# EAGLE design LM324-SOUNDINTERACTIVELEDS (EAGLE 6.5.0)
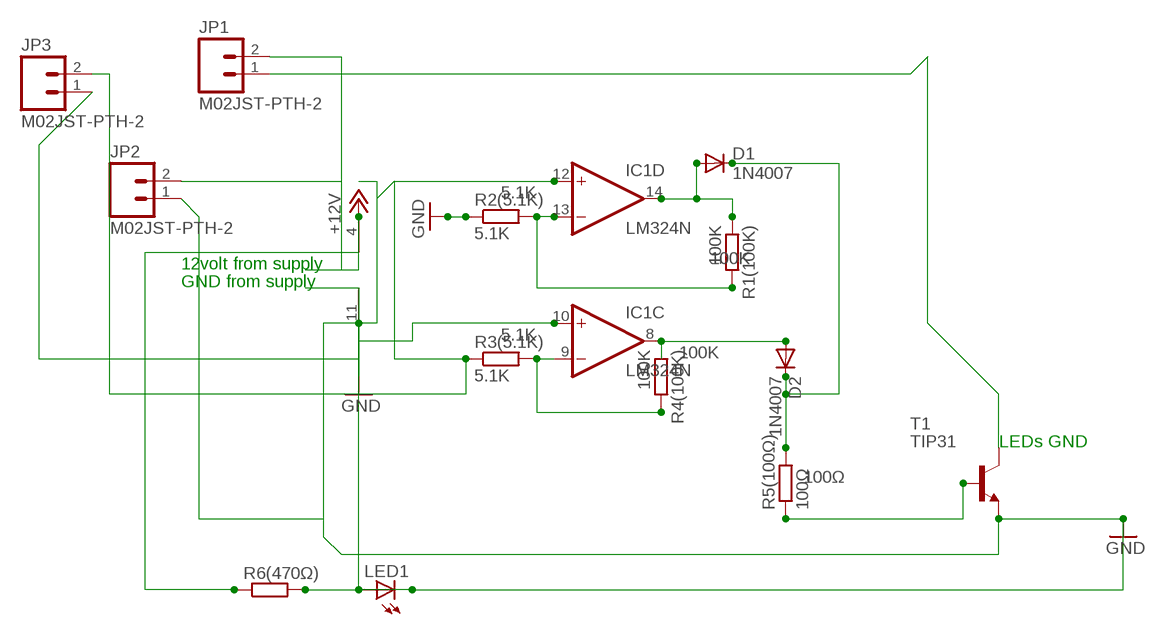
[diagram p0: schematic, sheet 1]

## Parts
D1  1N4007  1N4004  [DO41-10]
D2  1N4007  1N4004  [DO41-10]
IC1  LM324N  [DIL14]
JP1  M02JST-PTH-2  [JST-2-PTH]
JP2  M02JST-PTH-2  [JST-2-PTH]
JP3  M02JST-PTH-2  [JST-2-PTH]
LED1  LED5MM  [LED5MM]
R1(100K)  100K  R-EU_0204/7  [0204/7]
R2(5.1K)  5.1K  R-EU_0204/7  [0204/7]
R3(5.1K)  5.1K  R-EU_0204/7  [0204/7]
R4(100K)  100K  R-EU_0204/7  [0204/7]
R5(100Ω)  100Ω  R-EU_0204/7  [0204/7]
R6(470Ω)  R-EU_0204/7  [0204/7]
T1  TIP31  [TO220]

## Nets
+12V: IC1.4(P:V+) JP1.2 JP2.2 R6(470Ω).1
GND: IC1.10(C:+IN) IC1.11(P:V-) JP2.1 JP3.1 LED1.K(C) R2(5.1K).1 T1.3(E)
N$1: D1.A IC1.14(D:OUT) R1(100K).1
N$2: IC1.13(D:-IN) R1(100K).2 R2(5.1K).2
N$3: IC1.12(D:+IN) JP3.2 R3(5.1K).1
N$4: IC1.9(C:-IN) R3(5.1K).2 R4(100K).2
N$5: D2.A IC1.8(C:OUT) R4(100K).1
N$6: LED1.A R6(470Ω).2
N$7: D1.C D2.C R5(100Ω).2
N$8: JP1.1 T1.2(C)
N$11: R5(100Ω).1 T1.1(B)
Unconnected: IC1.1(A:OUT) IC1.2(A:-IN) IC1.3(A:+IN) IC1.5(B:+IN) IC1.6(B:-IN) IC1.7(B:OUT)

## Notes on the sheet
- 12volt from supply
- GND from supply
- LEDs GND

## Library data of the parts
D1 D2 = diode:1N4004: DIODE
IC1 = Unknown-5:LM324: OP AMP
JP1-JP3 = SparkFun-Connectors:M02: Standard 2-pin 0.1" header. Use with
LED1 = adafruit:LED: LED
R1(100K) = resistor:R-EU_: RESISTOR, European symbol; R1: 100K
R2(5.1K) R3(5.1K) = resistor:R-EU_: RESISTOR, European symbol; R2: 5.1K
R4(100K) = resistor:R-EU_: RESISTOR, European symbol; R4: 100K
R5(100Ω) = resistor:R-EU_: RESISTOR, European symbol; R5: 100Ω
R6(470Ω) = resistor:R-EU_: RESISTOR, European symbol
T1 = transistor:TIP31: NPN Transistor Medium Power Linear Switching Applications Source: http://onsemi.com

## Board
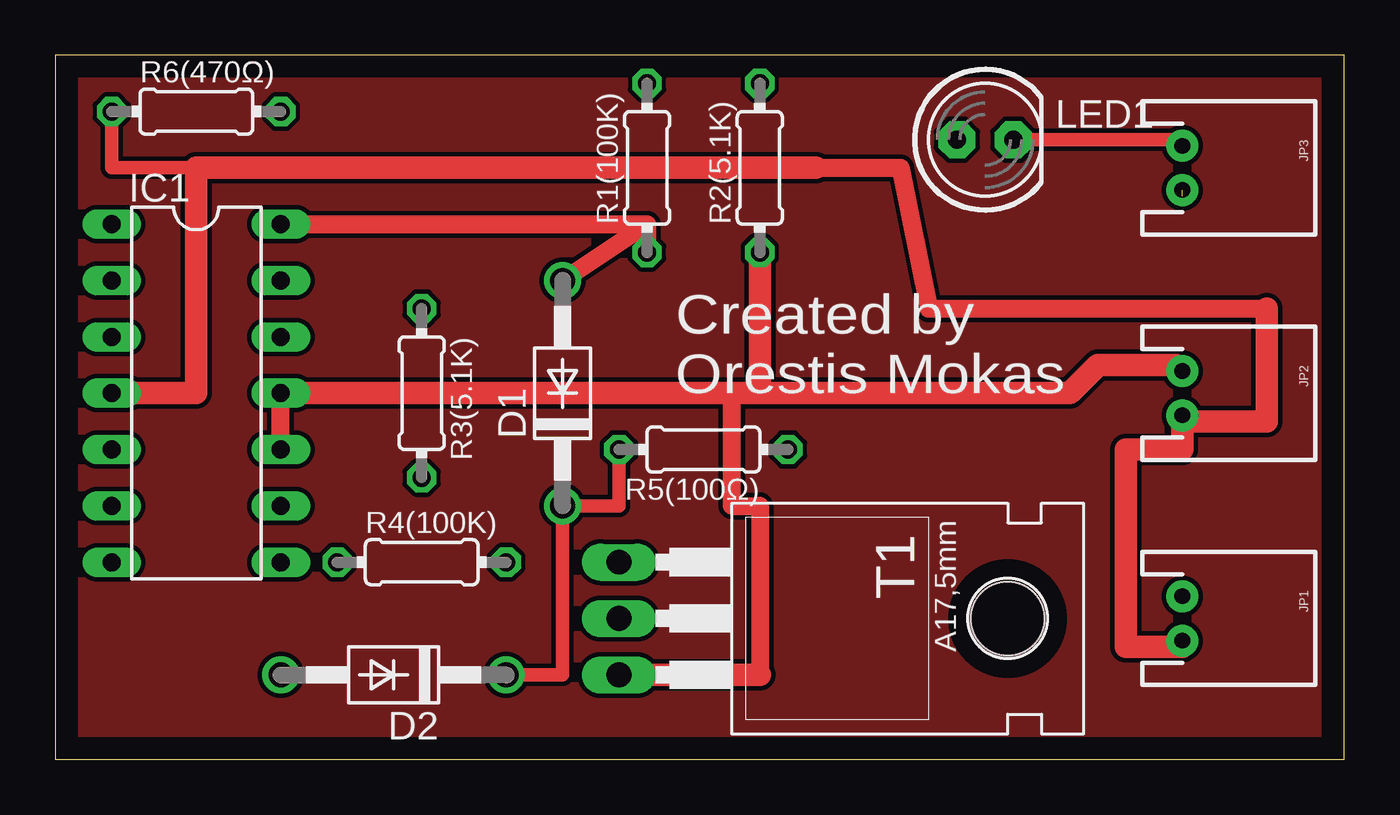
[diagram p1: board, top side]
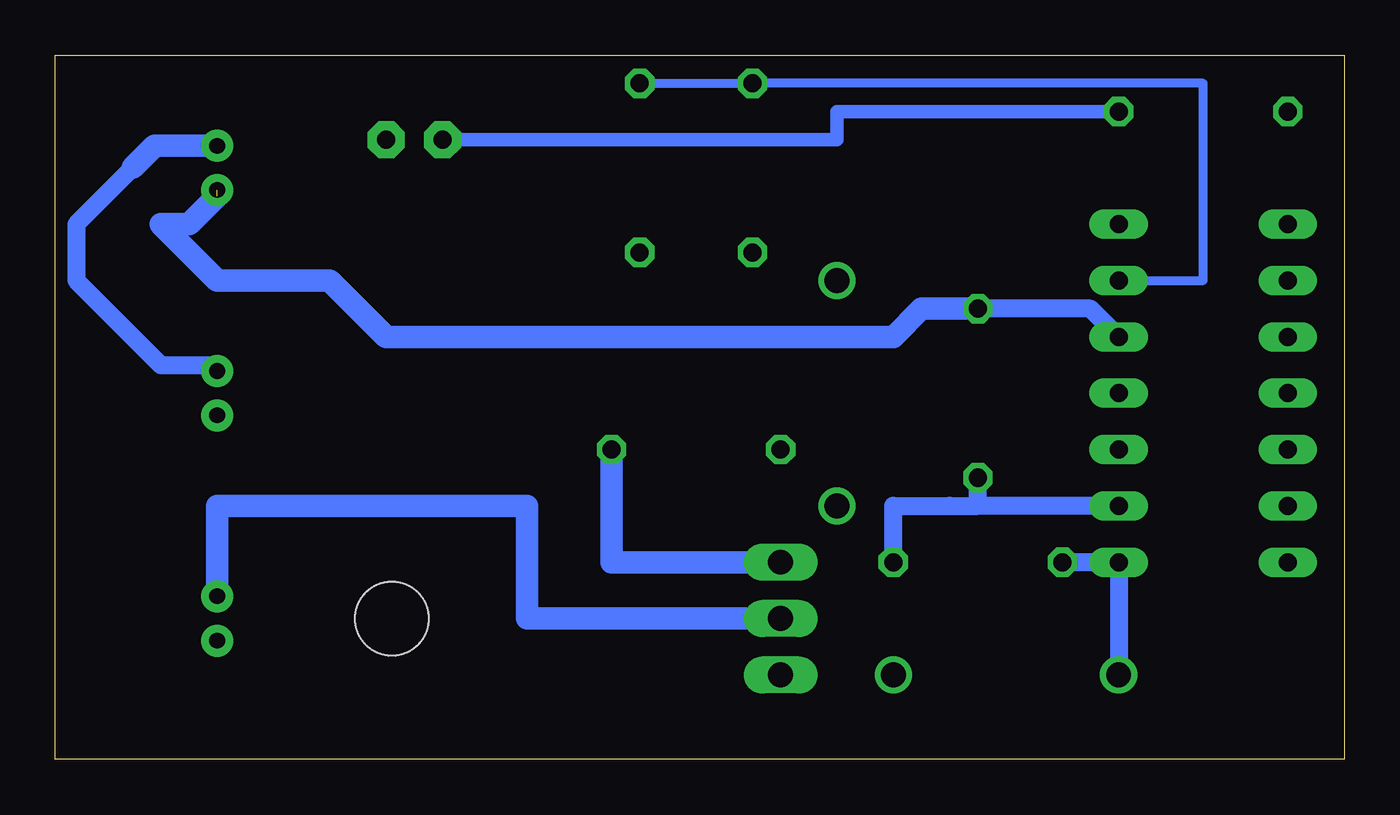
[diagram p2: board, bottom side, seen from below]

Size 58.09 x 31.74 mm. Coordinates in mm from the lower left corner, seen from the top.
Outline: 0,0 58.09,0 58.09,31.74 0,31.74 0,0
Copper layers (1*16): Top 0.035mm / dielectric 1.5mm / Bottom 0.035mm
Design rules "default": minimum track width 10mil, minimum drill 24mil, track to track 8mil, track to pad 8mil, pad to pad 8mil, via to via 8mil, smd to smd 8mil, copper to edge 40mil, drill to drill 8mil, minimum pad ring 10mil, minimum via ring 8mil, stop-mask expansion 4mil, vias tented up to drill 0mil, thermal gap 10mil

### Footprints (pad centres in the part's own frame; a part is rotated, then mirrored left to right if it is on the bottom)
DO41-10 = drill 1.118: A 5.08,0; C -5.08,0
DIL14 = drill 0.813 long: 1 -7.62,-3.81; 2 -5.08,-3.81; 3 -2.54,-3.81; 4 0,-3.81; 5 2.54,-3.81; 6 5.08,-3.81; 7 7.62,-3.81; 8 7.62,3.81; 9 5.08,3.81; 10 2.54,3.81; 11 0,3.81; 12 -2.54,3.81; 13 -5.08,3.81; 14 -7.62,3.81
JST-2-PTH = drill 0.7 pad 1.448: 1 -1,0; 2 1,0
LED5MM = drill 0.813 pad 1.676 octagon: A -1.27,0; K 1.27,0
0204/7 = drill 0.813 octagon: 1 -3.81,0; 2 3.81,0
TO220 = drill 1.118 long: 1 -2.54,-6.35; 2 0,-6.35; 3 2.54,-6.35 | hole 3.302: 0,11.176

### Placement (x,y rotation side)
D1  22.86,16.51 90 top
D2  15.24,3.81 180 top
IC1  6.35,16.51 270 top
JP1  50.8,6.35 270 top
JP2  50.8,16.51 270 top
JP3  50.8,26.67 270 top
LED1  41.91,27.94 0 top
R1(100K)  26.67,26.67 90 top
R2(5.1K)  31.75,26.67 90 top
R3(5.1K)  16.51,16.51 270 top
R4(100K)  16.51,8.89 0 top
R5(100Ω)  29.21,13.97 180 top
R6(470Ω)  6.35,29.21 0 top
T1  31.75,6.35 270 top

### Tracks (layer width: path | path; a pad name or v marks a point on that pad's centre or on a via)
+12V
  Top 0.61: R6(470Ω).1 2.54,26.67 6.35,26.67
  Top 0.813: 34.29,26.67 38.1,26.67 39.37,20.32 54.61,20.32
  Top 1.016: JP1.2 50.8,5.08 48.26,5.08 48.26,13.97 50.8,13.97 JP2.2 50.8,15.24 54.61,15.24 54.61,20.32 | 34.29,26.67 6.35,26.67 6.35,16.51 IC1.4
GND
  Top 0.61: LED1.K 50.8,27.94 JP3.1
  Top 0.813: IC1.10 IC1.11 | 30.48,16.51 30.48,11.43 31.75,11.43 31.75,3.81
  Top 1.016: IC1.11 30.48,16.51 31.75,16.51 | 31.75,16.51 R2(5.1K).1 | T1.3 31.75,3.81 | 31.75,16.51 45.72,16.51 46.99,17.78 50.53,17.78 JP2.1
  Bottom 0.813: 54.61,26.67 57.15,24.13 57.15,21.59 53.34,17.78 51.07,17.78 JP2.1
  Bottom 1.016: JP3.1 53.61,27.67 54.61,26.67
N$1
  Top 0.813: IC1.14 26.67,24.13 | 26.67,24.13 R1(100K).1 | D1.A 26.67,24.13
N$2
  Bottom 0.406: R2(5.1K).2 R1(100K).2 6.35,30.48 6.35,21.59 IC1.13
N$3  (1 unrouted)
  Bottom 0.813: IC1.12 11.43,20.32 R3(5.1K).1
  Bottom 1.016: R3(5.1K).1 19.05,20.32 20.32,19.05 43.18,19.05 45.72,21.59 50.8,21.59 53.34,24.13 52.07,24.13 50.8,25.4
N$4
  Bottom 0.813: R4(100K).2 20.32,11.43 17.78,11.43 16.51,11.43 | 16.51,11.43 R3(5.1K).2 | IC1.9 16.51,11.43
N$5
  Bottom 0.813: R4(100K).1 IC1.8 D2.A
N$6
  Bottom 0.61: R6(470Ω).2 22.86,29.21 22.86,27.94 LED1.A
N$7
  Top 0.61: D2.C 22.86,3.81 D1.C 25.4,11.43 R5(100Ω).2
N$8
  Bottom 1.016: T1.2 36.83,6.35 36.83,11.43 50.8,11.43 JP1.1
N$9
  pour Top: 0,0 0,31.75 58.42,31.75 58.42,0
N$11
  Bottom 1.016: T1.1 26.67,8.89 27.94,8.89 33.02,8.89 R5(100Ω).1

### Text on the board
tNames: Created by / Orestis Mokas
